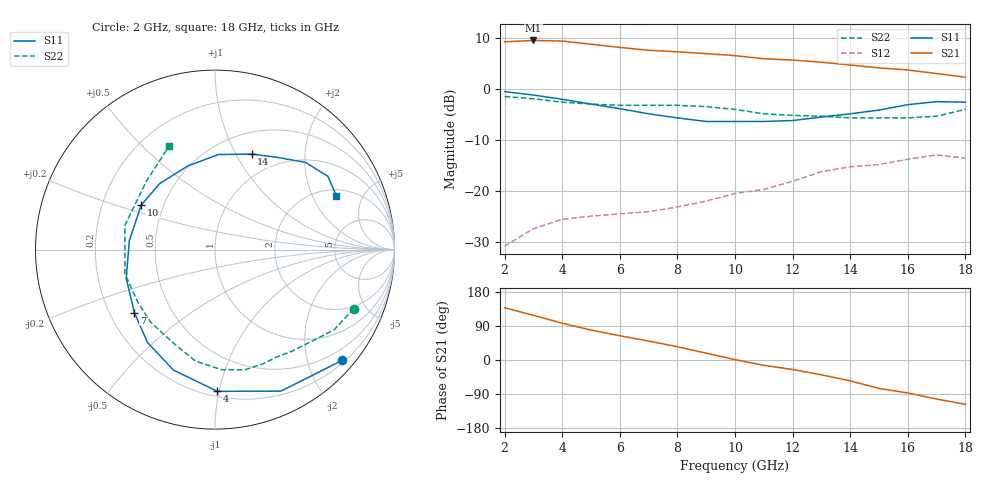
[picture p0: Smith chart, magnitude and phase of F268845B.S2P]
!ATF-26884
!S-PARAMETERS at Vds=5V  Id=30mA.  LAST UPDATED 07-22-92
# ghz s ma r 50
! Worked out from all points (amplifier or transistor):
!   17 points, 2 GHz to 18 GHz, reference 50 ohm
!   highest |S21| = 9.5 dB at 3 GHz (marker M1)
!   |S21| within 3 dB of that: start of sweep to 10.05 GHz
!   unconditionally stable (mu >= 1): 6.074 GHz to 9.684 GHz; 10.14 GHz to 11.7 GHz
!   at 4 GHz: K = 0.63, MSG = 17.4 dB, |S12| = -25.5 dB
!   at 10 GHz: K = 0.98, MSG = 13.5 dB, |S12| = -20.4 dB
!   at 18 GHz: K = 0.41, MSG = 7.9 dB, |S12| = -13.6 dB
!   S11 on the Smith chart (normalised r, x): 2 GHz: 0.25, -2.65; 4 GHz: 0.24, -0.99; 7 GHz: 0.30, -0.32; 10 GHz: 0.37, +0.24; 14 GHz: 0.74, +1.16; 18 GHz: 2.31, +3.08
2  0.94 -41.0  2.88 138.0  0.029 65.0  0.84 -23.0
3  0.87 -65.0  2.97 118.0  0.043 51.0  0.8 -34.0
4  0.79 -89.0  2.93 97.0  0.053 40.0  0.74 -44.0
5  0.71 -109.0  2.73 79.0  0.057 35.0  0.71 -53.0
6  0.64 -126.0  2.54 64.0  0.06 33.0  0.69 -60.0
7  0.57 -142.0  2.38 50.0  0.063 31.0  0.69 -67.0
8  0.52 -162.0  2.3 35.0  0.07 30.0  0.69 -76.0
9  0.48 174.0  2.21 18.0  0.08 28.0  0.67 -87.0
10  0.48 149.0  2.11 1.0  0.095 24.0  0.63 -100.0
11  0.48 130.0  1.97 -14.0  0.104 22.0  0.57 -114.0
12  0.49 108.0  1.91 -25.0  0.125 20.0  0.55 -122.0
13  0.53 88.0  1.82 -39.0  0.155 18.0  0.54 -132.0
14  0.57 69.0  1.71 -55.0  0.173 5.0  0.52 -146.0
15  0.62 56.0  1.6 -75.0  0.182 -1.0  0.52 -165.0
16  0.7 44.0  1.53 -87.0  0.205 -16.0  0.52 165.0
17  0.75 33.0  1.41 -103.0  0.226 -28.0  0.54 135.0
18  0.74 24.0  1.3 -117.0  0.21 -44.0  0.63 114.0
